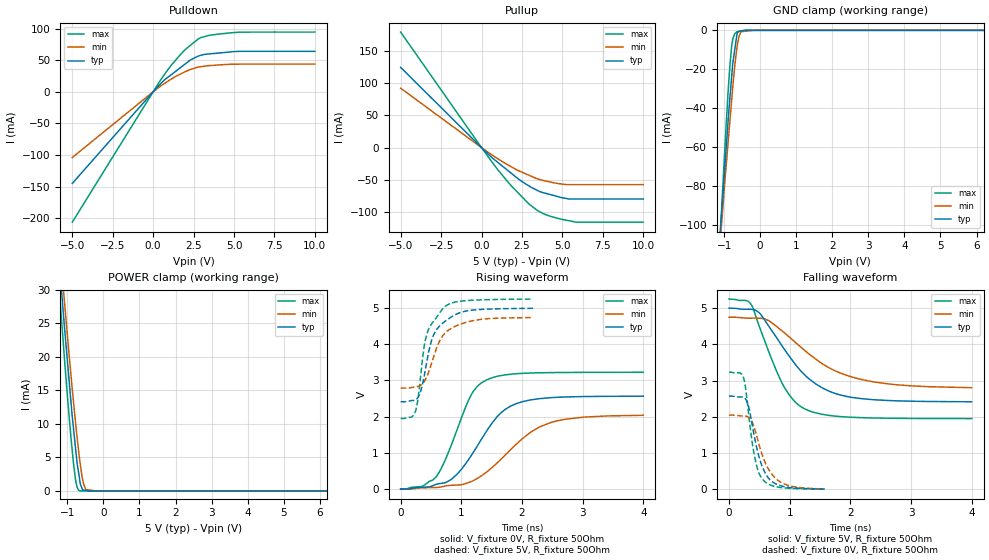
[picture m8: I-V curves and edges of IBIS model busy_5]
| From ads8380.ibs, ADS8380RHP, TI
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|   busy_5 Model
[Model]   busy_5
Model_type   3-state
Polarity   Non-Inverting
Vmeas = 2.5
Vref = 2.5
Cref = 10pF
Rref = 50
|   typ   min   max
|   (nom PVT)   (fast PVT)   (slow PVT)
|C_comp from frequency sweep method (F=1MHz)
|C_comp   2.602e-12   2.596e-12   2.649e-12
|ON state : BUFFER OUTPUT TURNED HIGH
|C_comp   2.602e-12   2.596e-12   2.649e-12
|OFF state: BUFFER IN HIGH IMPEDANCE
|C_comp   2.720e-12   2.612e-12   2.807e-12
|C_comp from LC tank measurement(L=1nH)
C_comp   6.368e-13   6.190e-13   6.617e-13
|Resonant Frequency(Hz)   6.320e+09   6.380e+09   6.200e+09
|C_comp   6.348e-13   6.229e-13   6.596e-13
|ON state : BUFFER OUTPUT TURNED HIGH
|Resonant Frequency(Hz)   6.320e+09   6.380e+09   6.200e+09
|C_comp   6.348e-13   6.229e-13   6.596e-13
|OFF state: BUFFER IN HIGH IMPEDANCE
|Resonant Frequency(Hz)   6.310e+09   6.400e+09   6.190e+09
|C_comp   6.368e-13   6.190e-13   6.617e-13
[Voltage Range]   5   4.75   5.25
[Temperature Range]   35   95   -40
[Pullup Reference]   5   4.75   5.25
[Pulldown Reference]   0   0   0
[Power Clamp Reference]   5   4.75   5.25
[GND Clamp Reference]   0   0   0
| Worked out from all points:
|   slope of the pulldown table from 0 to 0.75 V, typ, clamps not added: 38 ohm
|   slope of the pullup table from 0 to 0.75 V, typ, clamps not added: 42.3 ohm
|   GND clamp passes 1 mA (typ) near -0.62 V on its own axis
|   POWER clamp passes 1 mA (typ) near -0.64 V on its own axis
|   falling waveform, V_fixture 5V, R_fixture 50Ohm: 20-80 % time 748ps typ, 977ps min, 512ps max; typ from 5 V to 2.42 V
|   rising waveform, V_fixture 0V, R_fixture 50Ohm: 20-80 % time 638ps typ, 838ps min, 467ps max; typ from 0 V to 2.56 V
|   rising waveform, V_fixture 5V, R_fixture 50Ohm: 20-80 % time 262ps typ, 308ps min, 226ps max; typ from 2.41 V to 4.99 V
|   falling waveform, V_fixture 0V, R_fixture 50Ohm: 20-80 % time 225ps typ, 280ps min, 167ps max; typ from 2.57 V to 0.012 V
[Pulldown]
|   Voltage   I(typ)   I(min)   I(max)
-5V       -144.9mA   -103.9mA   -206.2mA
425.3mV   11.75mA    8.409mA    17.37mA
924mV     23.18mA    16.95mA    35.51mA
1.596V    36.42mA    27.07mA    56.31mA
2.011V    44.59mA    32.13mA    67.4mA
2.27V     49.69mA    34.93mA    72.81mA
2.793V    56.42mA    39.22mA    83.73mA
3.46V     59.87mA    41.37mA    89.24mA
5.318V    63.92mA    43.76mA    94.26mA
10V       63.98mA    43.79mA    94.45mA
[GND Clamp]
|   Voltage   I(typ)   I(min)   I(max)
-5V       -1.317A    -1.15A     -1.875A
-1.088V   -97.97mA   -103.5mA   -99.09mA
-1.045V   -86.82mA   -93.3mA    -83.33mA
-955.5mV  -63.76mA   -72.34mA   -52.55mA
-834.7mV  -33.62mA   -45.54mA   -17mA
-792.7mV  -24.22mA   -36.22mA   -8.58mA
-756mV    -16.39mA   -28.15mA   -4.121mA
-640.5mV  -1.642mA   -8.441mA   -729.4uA
-584.3mV  -563.8uA   -2.825mA   -508.2uA
-532mV    -390.4uA   -718.3uA   -302.8uA
-190mV    0A         -32.43nA   -2.902uA
10V       0A         0A         0A
[Pullup]
|   Voltage   I(typ)   I(min)   I(max)
-5V       124.5mA    92.27mA    179.4mA
115.6fV   -79.82pA   -98.94pA   -72.32pA
924mV     -21.25mA   -15.91mA   -31.72mA
1.822V    -39.47mA   -29.55mA   -58.86mA
2.27V     -48.57mA   -35.64mA   -70.41mA
2.94V     -59.62mA   -42.98mA   -87.67mA
3.465V    -66.64mA   -48.5mA    -97.83mA
4.058V    -71.6mA    -52.31mA   -104.9mA
5.405V    -79.77mA   -57.54mA   -113.6mA
5.87V     -79.77mA   -57.54mA   -115.8mA
10V       -79.77mA   -57.54mA   -115.8mA
[POWER Clamp]
|   Voltage   I(typ)   I(min)   I(max)
-5V       555.6mA    444.8mA    819.5mA
-1.306V   39.53mA    42.72mA    35.96mA
-1.088V   24.91mA    28.69mA    20.27mA
-971.2mV  17.69mA    21.51mA    12.38mA
-829.5mV  9.28mA     13.29mA    4.118mA
-771.8mV  6.287mA    10.14mA    1.651mA
-687.7mV  2.707mA    5.963mA    93.45uA
-640mV    1.014mA    3.922mA    9.836uA
-546.3mV  125.6uA    929.3uA    1.201uA
-484.5mV  66.71uA    197.5uA    1.066uA
-190mV    0A         22.35nA    418.1nA
10V       0A         0A         0A
[Ramp]
R_load = 50
|   typ   min   max
dV/dt_r   1.53909/6.3631e-10   1.22282/8.30702e-10   1.93489/4.65884e-10
dV/dt_f   1.54923/7.47558e-10   1.16617/9.76263e-10   1.977/5.12193e-10
[Falling Waveform]
V_fixture = 5V
V_fixture_min = 4.75V
V_fixture_max = 5.25V
R_fixture = 50Ohm
|   Time   V(typ)   V(min)   V(max)
0s        5V         4.75V      5.25V
362ps     4.969V     4.723V     5.109V
518ps     4.837V     4.72V      4.409V
866ps     3.98V      4.384V     2.959V
1.054ns   3.534V     4.115V     2.479V
1.246ns   3.16V      3.836V     2.223V
1.69ns    2.683V     3.319V     2.034V
2.194ns   2.503V     3.029V     1.979V
2.992ns   2.434V     2.858V     1.959V
3.998ns   2.418V     2.806V     1.955V
[Rising Waveform]
V_fixture = 0V
V_fixture_min = 0V
V_fixture_max = 0V
R_fixture = 50Ohm
|   Time   V(typ)   V(min)   V(max)
0s        1.729nV    3.388nV    1.523nV
354ps     51.69mV    37.14mV    78.35mV
586ps     134.3mV    45.86mV    342.7mV
844ps     281.7mV    108.1mV    1.254V
1.15ns    893.4mV    201.1mV    2.559V
1.41ns    1.586V     463.7mV    3.009V
1.798ns   2.278V     1.066V     3.168V
2.146ns   2.463V     1.575V     3.204V
2.474ns   2.524V     1.838V     3.216V
3.998ns   2.565V     2.038V     3.225V
[Rising Waveform]
V_fixture = 5V
V_fixture_min = 4.75V
V_fixture_max = 5.25V
R_fixture = 50Ohm
|   Time   V(typ)   V(min)   V(max)
0s        2.412V     2.79V      1.953V
238ps     2.458V     2.822V     2.123V
282ps     2.523V     2.833V     2.444V
328ps     2.692V     2.863V     3.097V
382ps     3.065V     2.954V     3.876V
436ps     3.558V     3.121V     4.3V
548ps     4.275V     3.675V     4.645V
736ps     4.635V     4.313V     5.045V
1.176ns   4.939V     4.644V     5.212V
2.18ns    4.99V      4.735V     5.245V
[Falling Waveform]
V_fixture = 0V
V_fixture_min = 0V
V_fixture_max = 0V
R_fixture = 50Ohm
|   Time   V(typ)   V(min)   V(max)
0s        2.57V      2.048V     3.227V
180ps     2.552V     2.031V     3.216V
244ps     2.537V     2.028V     3.059V
316ps     2.331V     1.997V     2.182V
410ps     1.527V     1.732V     1.012V
472ps     1.041V     1.376V     554.9mV
546ps     639.3mV    958mV      294.5mV
666ps     283.9mV    521.5mV    135.3mV
860ps     99.11mV    192mV      52.96mV
1.576ns   11.78mV    16.3mV     8.97mV
